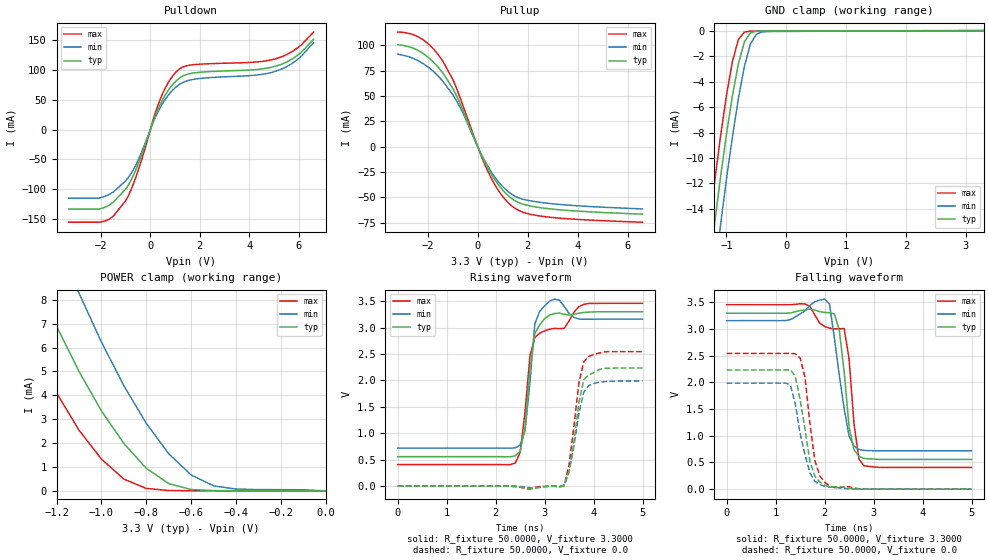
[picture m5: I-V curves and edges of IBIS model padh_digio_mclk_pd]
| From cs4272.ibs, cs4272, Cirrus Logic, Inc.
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|   Model mclkp
[Model]  padh_digio_mclk_pd
Model_type I/O
Polarity   Non-Inverting
Enable   Active-High
Vinl =   0.8000V
Vinh =   2.0000V
C_comp   5.0000pF   5.0000pF   5.0000pF
[Temperature Range]   25.0000   85.0000   -40.0000
[Voltage Range]   3.3000V   3.0000V   3.6000V
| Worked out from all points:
|   slope of the pulldown table from 0 to 0.495 V, typ, clamps not added: 9.87 ohm
|   slope of the pullup table from 0 to 0.495 V, typ, clamps not added: 19.8 ohm
|   GND clamp passes 1 mA (typ) near -0.71 V on its own axis
|   POWER clamp passes 1 mA (typ) near -0.81 V on its own axis
|   rising waveform, R_fixture 50.0000, V_fixture 3.3000: 20-80 % time 181ps typ, 146ps min, 295ps max; typ from 0.557 V to 3.3 V
|   rising waveform, R_fixture 50.0000, V_fixture 0.0: 20-80 % time 218ps typ, 228ps min, 207ps max; typ from 0 V to 2.23 V
|   falling waveform, R_fixture 50.0000, V_fixture 3.3000: 20-80 % time 185ps typ, 235ps min, 203ps max; typ from 3.3 V to 0.557 V
|   falling waveform, R_fixture 50.0000, V_fixture 0.0: 20-80 % time 250ps typ, 270ps min, 204ps max; typ from 2.23 V to 0 V
[Pulldown]
|Voltage   I(typ)   I(min)   I(max)
-3.3V     -133.6mA   -115.4mA   -155.6mA
-2.1V     -133.6mA   -115.4mA   -155.6mA
-1.7V     -127.8mA   -109.7mA   -151.4mA
-1V       -100mA     -86.22mA   -119.6mA
-500mV    -58.64mA   -51.91mA   -69.38mA
400mV     42.39mA    37.02mA    51.17mA
800mV     70.37mA    61.68mA    84mA
1.2V      87.05mA    76.46mA    102.6mA
1.8V      95.27mA    84.7mA     109.2mA
5.1V      106.8mA    98.32mA    119.3mA
5.9V      123.2mA    116.1mA    135.5mA
6.6V      151.5mA    146mA      163.7mA
[Pullup]
|Voltage   I(typ)   I(min)   I(max)
-3.2V     100.5mA    91.23mA    113mA
-2.2V     92.16mA    82.21mA    105.7mA
-1.4V     72.9mA     64.63mA    84.58mA
-1V       57.56mA    51.29mA    66.47mA
-700mV    42.4mA     38.53mA    48.01mA
100mV     -5.682mA   -5.222mA   -6.579mA
400mV     -20.84mA   -19.16mA   -24.02mA
900mV     -40mA      -36.76mA   -45.85mA
1.4V      -51.95mA   -47.64mA   -59.29mA
1.9V      -57.48mA   -52.52mA   -65.51mA
2.7V      -60.95mA   -55.7mA    -69.25mA
6.6V      -66.7mA    -61.6mA    -74.67mA
[GND_clamp]
|Voltage   I(typ)   I(min)   I(max)
-3.3V     -106.5mA   -109mA     -107.1mA
-1.3V     -19.2mA    -23.22mA   -15.95mA
-1.2V     -15.29mA   -19.2mA    -12mA
-1.1V     -11.58mA   -15.36mA   -8.342mA
-1V       -8.152mA   -11.7mA    -5.094mA
-900mV    -5.127mA   -8.36mA    -2.41mA
-800mV    -2.581mA   -5.332mA   -671.1uA
-700mV    -859.1uA   -2.795mA   -85.29uA
-600mV    -150.6uA   -1.045mA   -9.486uA
-500mV    -16.29uA   -251.8uA   -4.509uA
-400mV    -3.582uA   -68.44uA   -3.47uA
3.3V      6.714uA    56.14uA    8.702uA
[POWER_clamp]
|Voltage   I(typ)   I(min)   I(max)
-3.3V     67.56mA    73.97mA    64.02mA
-1.4V     11.24mA    15.44mA    7.981mA
-1.3V     8.978mA    12.91mA    5.927mA
-1.2V     6.891mA    10.51mA    4.102mA
-1.1V     5.004mA    8.28mA     2.545mA
-1V       3.352mA    6.233mA    1.334mA
-900mV    1.988mA    4.403mA    495.9uA
-800mV    946uA      2.827mA    104.5uA
-700mV    305.7uA    1.557mA    18.2uA
-600mV    58.51uA    667.2uA    9.264uA
-400mV    7.044uA    77.88uA    8.713uA
0V        0A         0A         0A
[Ramp]
| variable   typ   min   max
dV/dt_r  1.3410/0.2374n   1.0956/0.2946n   1.6002/0.1795n
dV/dt_f  1.6454/0.1598n   1.4009/0.2014n   1.8901/0.1132n
R_load = 50.0000
[Rising Waveform]
R_fixture= 50.0000
V_fixture= 3.3000
V_fixture_min= 3.6000
V_fixture_max= 3.0000
|time   V(typ)   V(min)   V(max)
0s        556.7mV    720.1mV    406.8mV
2.4ns     572.7mV    723.4mV    435.4mV
2.5ns     660.9mV    775.7mV    638mV
2.6ns     1.113V     1.041V     1.401V
2.7ns     2.205V     1.956V     2.464V
2.8ns     2.889V     3.071V     2.81V
3ns       3.169V     3.411V     2.936V
3.4ns     3.251V     3.402V     2.985V
3.8ns     3.286V     3.156V     3.438V
5ns       3.299V     3.16V      3.458V
[Rising Waveform]
R_fixture= 50.0000
V_fixture= 0.0
|time   V(typ)   V(min)   V(max)
0s        0V         252.7uV    0V
2.7ns     -53.75mV   -32.81mV   -58.04mV
3.4ns     30uV       26.29mV    11.8mV
3.5ns     277.6mV    274.5mV    406.6mV
3.6ns     842mV      761.6mV    1.145V
3.7ns     1.583V     1.38V      1.952V
3.8ns     2.014V     1.774V     2.353V
3.9ns     2.105V     1.902V     2.452V
4.2ns     2.227V     1.974V     2.537V
5ns       2.235V     1.988V     2.544V
[Falling Waveform]
R_fixture= 50.0000
V_fixture= 3.3000
V_fixture_min= 3.6000
V_fixture_max= 3.0000
|time   V(typ)   V(min)   V(max)
0s        3.299V     3.159V     3.458V
1.6ns     3.361V     3.342V     3.473V
2ns       3.313V     3.564V     3.051V
2.1ns     3.307V     3.468V     3.019V
2.2ns     3.284V     2.828V     3.006V
2.4ns     2.19V      1.506V     3.011V
2.5ns     1.163V     988.2mV    2.439V
2.6ns     741.4mV    808.6mV    1.226V
2.8ns     577.5mV    727.1mV    440.8mV
5ns       556.7mV    719.7mV    406.8mV
[Falling Waveform]
R_fixture= 50.0000
V_fixture= 0.0
|time   V(typ)   V(min)   V(max)
0s        2.235V     1.987V     2.544V
1.3ns     2.236V     1.956V     2.545V
1.4ns     2.12V      1.607V     2.54V
1.5ns     1.678V     1.041V     2.46V
1.6ns     1.121V     640.4mV    2.092V
1.7ns     513.1mV    306mV      1.226V
1.8ns     246.4mV    148.3mV    539.8mV
1.9ns     135mV      84.13mV    250.8mV
2.1ns     41.89mV    39.63mV    63.46mV
5ns       -10.69uV   0V         1.925uV
